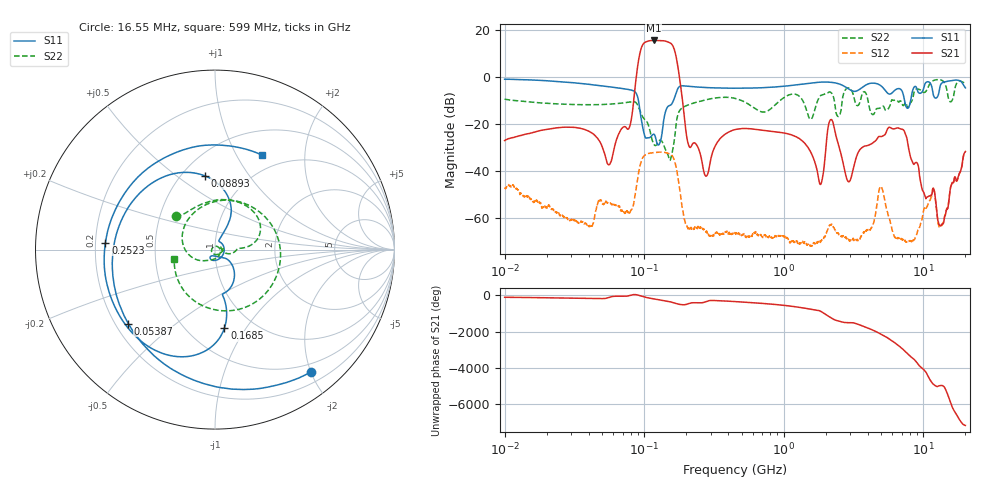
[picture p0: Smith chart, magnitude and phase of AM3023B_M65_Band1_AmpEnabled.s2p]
!Agilent Technologies,E8364B,MY43040894,A.07.50.67
!Agilent E8364B: A.07.50.67
!Date: Tuesday, October 27, 2020 10:52:09
!Correction: S11(Full 2 Port(1,2))
!S21(Full 2 Port(1,2))
!S12(Full 2 Port(1,2))
!S22(Full 2 Port(1,2))
!S2P File: Measurements: S11, S21, S12, S22:Log Frequency Sweep
# Hz S  dB  R 50
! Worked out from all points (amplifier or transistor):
!   3201 points, 10 MHz to 20 GHz, reference 50 ohm
!   highest |S21| = 15.6 dB at 116.9 MHz (marker M1)
!   |S21| within 3 dB of that: 95.63 MHz to 162.4 MHz (66.78 MHz wide, 51.8 % of centre)
!   unconditionally stable (mu >= 1): start of sweep to end of sweep
!   at 35.47 MHz: K = 3206.04, MAG = -18.2 dB, |S12| = -61.6 dB
!   at 447.2 MHz: K = 7671.31, MAG = -19.9 dB, |S12| = -66.2 dB
!   at 20 GHz: K = 218.63, MAG = -26.3 dB, |S12| = -31.9 dB
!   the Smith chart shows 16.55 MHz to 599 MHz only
!   S11 on the Smith chart (normalised r, x): 16.55 MHz: 0.37, -2.00; 53.87 MHz: 0.25, -0.35; 88.93 MHz: 0.65, +0.64; 168.5 MHz: 0.74, -0.80; 252.3 MHz: 0.24, +0.03; 599 MHz: 0.80, +1.29
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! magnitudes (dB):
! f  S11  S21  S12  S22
! 10 MHz  -0.9  -27.0  -47.6  -9.3
! 16.55 MHz  -1.3  -23.3  -52.7  -10.8
! 35.55 MHz  -2.7  -21.9  -61.7  -11.7
! 53.87 MHz  -3.9  -36.1  -53.2  -11.5
! 78.6 MHz  -5.3  -21.1  -57.8  -10.6
! 88.93 MHz  -7.7  2.9  -44.8  -11.4
! 116.9 MHz  -24.3  15.6  -32.1  -28.4
! 126.1 MHz  -28.9  15.6  -31.9  -27.5
! 168.5 MHz  -7.1  9.3  -37.8  -21.1
! 205.7 MHz  -3.9  -27.9  -64.5  -11.8
! 252.3 MHz  -4.3  -32.7  -64.0  -10.2
! 447.2 MHz  -4.7  -22.3  -66.2  -9.0
! 599 MHz  -4.6  -22.0  -66.6  -12.7
! 1.59 GHz  -2.5  -32.9  -71.9  -17.5
! 1.851 GHz  -2.1  -45.3  -69.8  -7.7
! 2.196 GHz  -2.2  -18.1  -62.6  -6.7
! 2.934 GHz  -5.1  -44.5  -69.5  -4.6
! 4.948 GHz  -3.6  -25.3  -46.5  -13.0
! 5.639 GHz  -7.1  -21.4  -59.2  -13.2
! 11.72 GHz  -6.9  -47.3  -47.2  -1.5
! 13.32 GHz  -3.1  -63.2  -63.8  -1.1
! 20 GHz  -4.5  -31.6  -31.9  -2.6
